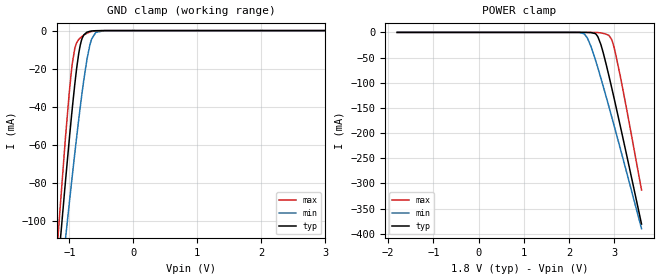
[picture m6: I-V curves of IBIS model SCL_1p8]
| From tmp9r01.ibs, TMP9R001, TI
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|   Model
[Model]   SCL_1p8
Model_type   Input
Vinl = 0.54
Vinh = 1.26
|   typ   min   max
C_comp   0.826pF   0.806pF   0.832pF
[Voltage Range]   1.8   1.7   2
[Temperature Range]   25   125   -40
[Power Clamp Reference]   1.8   1.7   2
[GND Clamp Reference]   0   0   0
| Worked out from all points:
|   GND clamp passes 1 mA (typ) near -0.73 V on its own axis
[GND Clamp]
|   Voltage   I(typ)   I(min)   I(max)
-1.8V     -380.9mA   -355.9mA   -412.7mA
-1.174V   -123mA     -145.8mA   -106.7mA
-1.147V   -112.4mA   -137.1mA   -94.28mA
-1.06V    -79.04mA   -109.3mA   -56.06mA
-1.001V   -57.12mA   -90.66mA   -32.45mA
-952.2mV  -40.21mA   -75.71mA   -16.96mA
-892.8mV  -21.82mA   -58mA      -6.966mA
-828mV    -7.476mA   -39.75mA   -3.822mA
-725.4mV  -849.8uA   -15.27mA   -1.427mA
-649.8mV  -213.3uA   -4.291mA   -466.1uA
-444.6mV  -2.216uA   -19.84uA   -3.303uA
3.6V      0A         0A         0A
[POWER Clamp]
|   Voltage   I(typ)   I(min)   I(max)
-1.8V     0A         0A         0A
2.25V     -2.566uA   -360.8uA   -11.62nA
2.336V    -20.33uA   -3.206mA   -93.55nA
2.401V    -81.96uA   -10.89mA   -841.8nA
2.59V     -3.262mA   -57.24mA   -141.7uA
2.633V    -8.339mA   -70.03mA   -344.8uA
2.741V    -36.63mA   -103.4mA   -1.718mA
2.882V    -87.24mA   -148.5mA   -6.141mA
2.941V    -110.2mA   -167.9mA   -14.27mA
2.984V    -127.3mA   -182.2mA   -26.68mA
3.141V    -190.4mA   -234.4mA   -91.73mA
3.6V      -380.9mA   -390.1mA   -313.2mA
